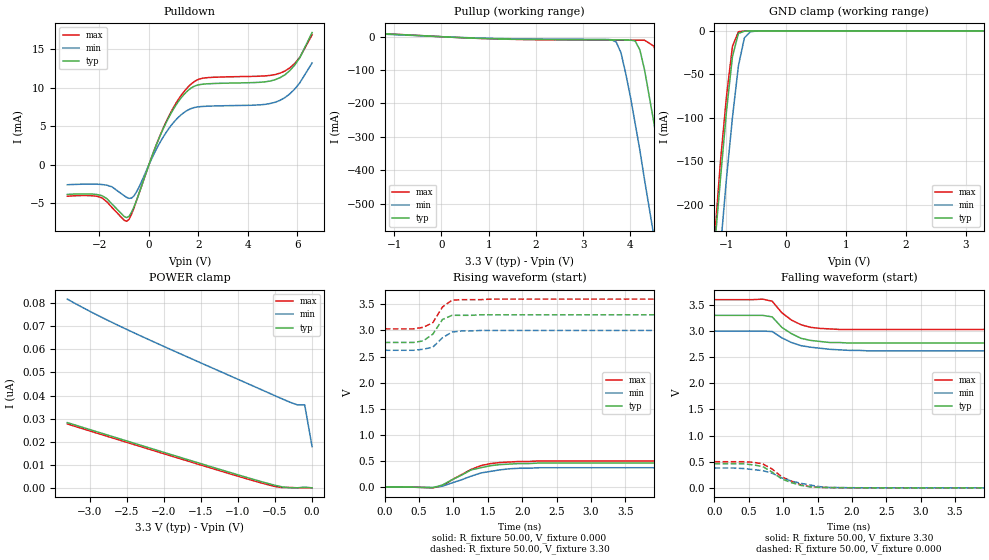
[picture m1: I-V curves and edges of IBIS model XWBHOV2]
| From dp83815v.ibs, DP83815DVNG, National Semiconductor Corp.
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|   Model XWBHOV2
[Model]   XWBHOV2
Model_type   I/O
Polarity   Non-Inverting
Enable   Active-High
Vinl =   0.80V
Vinh =   2.00V
Vmeas =   1.50V
Cref =  20.00pF
Rref = 100.00k
C_comp   5.00pF   5.00pF   5.00pF
[Temperature Range]   25.00   0.14k   0.000
[Voltage Range]   3.30V   3.00V   3.60V
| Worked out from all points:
|   slope of the pulldown table from 0 to 0.495 V, typ, clamps not added: 121 ohm
|   slope of the pullup table from 0 to 0.495 V, typ, clamps not added: 151 ohm
|   GND clamp passes 1 mA (typ) near -0.72 V on its own axis
|   rising waveform, R_fixture 50.00, V_fixture 0.000: 20-80 % time 480ps typ, 556ps min, 447ps max; typ from 0 V to 0.46 V
|   rising waveform, R_fixture 50.00, V_fixture 3.30: 20-80 % time 190ps typ, 209ps min, 188ps max; typ from 2.77 V to 3.3 V
|   falling waveform, R_fixture 50.00, V_fixture 3.30: 20-80 % time 342ps typ, 455ps min, 329ps max; typ from 3.3 V to 2.77 V
|   falling waveform, R_fixture 50.00, V_fixture 0.000: 20-80 % time 387ps typ, 531ps min, 394ps max; typ from 0.46 V to 0 V
[Pulldown]
| voltage   I(typ)   I(min)   I(max)
-3.3V     -3.85mA    -2.59mA    -4.08mA
-1.9V     -4.01mA    -2.56mA    -4.29mA
-900mV    -6.86mA    -4.23mA    -7.34mA
-700mV    -6.14mA    -4.32mA    -6.4mA
-500mV    -4.61mA    -3.51mA    -4.66mA
200mV     1.76mA     1.38mA     1.78mA
700mV     5.5mA      4.22mA     5.62mA
1.6V      9.71mA     7.15mA     10.17mA
2.2V      10.48mA    7.59mA     11.26mA
5.3V      11.31mA    8.37mA     11.9mA
5.9V      12.97mA    9.85mA     13.17mA
6.6V      17.18mA    13.23mA    16.89mA
[Pullup]
| voltage   I(typ)   I(min)   I(max)
-3.3V     4.05mA     2.54mA     8mA
3.6V      -9.56mA    -9.1mA     -10.26mA
3.8V      -9.66mA    -48.28mA   -10.35mA
4.1V      -12.7mA    -260mA     -10.46mA
4.2V      -39.42mA   -340mA     -10.52mA
4.3V      -100mA     -430mA     -10.66mA
4.5V      -260mA     -600mA     -28.5mA
4.7V      -440mA     -780mA     -160mA
4.9V      -610mA     -960mA     -330mA
5.1V      -800mA     -1.14A     -510mA
5.3V      -980mA     -1.32A     -690mA
6.6V      -2.17A     -2.51A     -1.88A
[GND_clamp]
| voltage   I(typ)   I(min)   I(max)
-3.3V     -2.16A     -2.23A     -2.15A
-1.2V     -250mA     -340mA     -240mA
-1.1V     -170mA     -250mA     -150mA
-1V       -92.65mA   -170mA     -75.94mA
-900mV    -29.63mA   -99.82mA   -17.91mA
-800mV    -2.96mA    -40.21mA   -1.07mA
-700mV    -420uA     -8.11mA    -140uA
-600mV    -130uA     -1.12mA    -21.94uA
-300mV    -130nA     -10.76uA   -3.69nA
3.3V      45.34pA    37.14nA    35.46pA
[POWER_clamp]
| voltage   I(typ)   I(min)   I(max)
-3.3V     28.29nA    81.75nA    27.7nA
-2.9V     24.32nA    74.9nA     23.73nA
-2.4V     19.37nA    67.15nA    18.78nA
-1.1V     6.65nA     48.46nA    6.05nA
-600mV    1.99nA     41.36nA    1.42nA
-400mV    440pA      38.52nA    140pA
-200mV    60.47pA    35.98nA    63.53pA
-100mV    360pA      35.98nA    40.81pA
0V        45.34pA    17.87nA    38.83pA
[Ramp]
| variable   typ   min   max
dV/dt_r   1.49/0.51n   1.28/0.62n   1.64/0.51n
dV/dt_f   1.58/0.40n   1.35/0.59n   1.73/0.38n
R_load = 0.50k
[Rising Waveform]
R_fixture = 50.00
V_fixture = 0.000
V_fixture_min = 0.000
V_fixture_max = 0.000
| time   V(typ)   V(min)   V(max)
0s        140uV      120uV      160uV
700ps     -12.03mV   -6.65mV    -15.65mV
840ps     40.13mV    16.49mV    22.02mV
980ps     140mV      80.7mV     140mV
1.26ns    330mV      210mV      340mV
1.4ns     370mV      270mV      410mV
1.54ns    410mV      300mV      450mV
1.68ns    430mV      330mV      470mV
1.96ns    450mV      360mV      490mV
7ns       460mV      370mV      500mV
[Rising Waveform]
R_fixture = 50.00
V_fixture = 3.30
V_fixture_min = 3.00
V_fixture_max = 3.60
| time   V(typ)   V(min)   V(max)
0s        2.77V      2.62V      3.03V
420ps     2.77V      2.62V      3.03V
560ps     2.8V       2.64V      3.06V
700ps     2.93V      2.68V      3.15V
840ps     3.21V      2.86V      3.45V
980ps     3.29V      2.97V      3.58V
1.12ns    3.29V      2.99V      3.59V
1.4ns     3.3V       3V         3.59V
1.54ns    3.3V       3V         3.6V
7ns       3.3V       3V         3.6V
[Falling Waveform]
R_fixture = 50.00
V_fixture = 3.30
V_fixture_min = 3.00
V_fixture_max = 3.60
| time   V(typ)   V(min)   V(max)
0s        3.3V       3V         3.6V
700ps     3.3V       3V         3.61V
840ps     3.27V      2.99V      3.57V
980ps     3.07V      2.87V      3.35V
1.12ns    2.95V      2.78V      3.21V
1.26ns    2.86V      2.72V      3.12V
1.4ns     2.82V      2.69V      3.07V
1.54ns    2.8V       2.67V      3.05V
2.24ns    2.77V      2.62V      3.03V
7ns       2.77V      2.62V      3.03V
[Falling Waveform]
R_fixture = 50.00
V_fixture = 0.000
V_fixture_min = 0.000
V_fixture_max = 0.000
| time   V(typ)   V(min)   V(max)
0s        460mV      380mV      500mV
420ps     460mV      370mV      500mV
700ps     410mV      330mV      460mV
840ps     300mV      280mV      360mV
980ps     170mV      190mV      210mV
1.12ns    100mV      130mV      130mV
1.26ns    46.09mV    86.8mV     57.09mV
1.54ns    8.95mV     21.44mV    8.82mV
2.24ns    750uV      1.34mV     670uV
7ns       -2.46uV    990nV      -1.26uV
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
